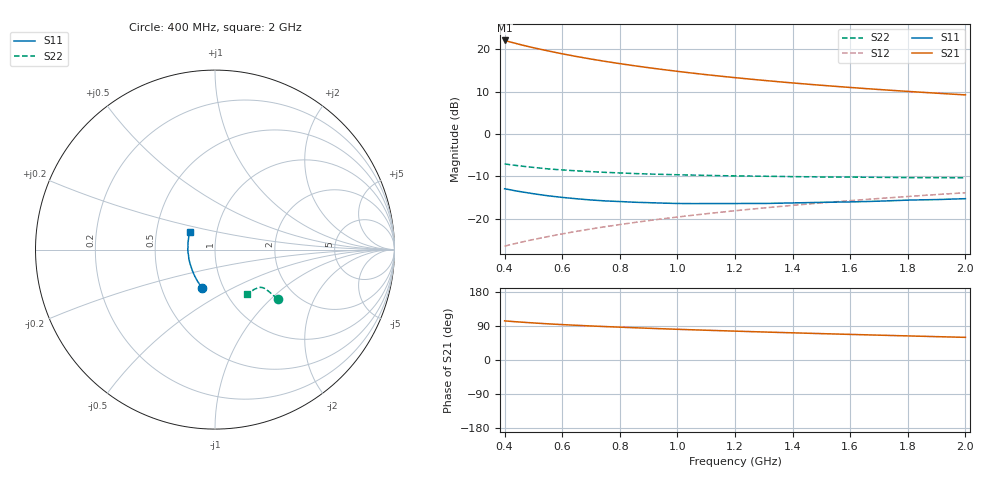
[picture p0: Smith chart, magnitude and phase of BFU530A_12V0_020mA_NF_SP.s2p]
! Filename:  P:\Prog\Test\Noise\ATS_data\Testdata_Net\06 Compressed Noise after Statistics\BFU530A_APG2013_33_A05_12p0V_020mA_NF_CM01_D.sf
! Date/Time: Tue 16/Apr/2013 15:11:00
! BFU530A_APG2013_33_A05_12p0V_1to25mA_NF_CM01_Bias7_R.sf
! Noise Parameter Data File
! BFU530A_APG2013_33_A05_12p0V_1to25mA_NF_CM01
! Date/time: Fri Apr 12 17:55:00 2013
! VAR V_out= 12.001000
! VAR I_out= 19.995000
! VAR V_in= 0.787500
! VAR I_in= 0.189800
! Device data file deembeded for feedlines and parallel
! Original file: \06 Compressed Noise after Statistics\BFU530A_APG2013_33_A05_12p0V_020mA_NF_CM01_R.sf
! Feed-files: PR017V01_150413_Feed1.s2p, PR017V01_150413_Feed2.s2p
! Parallel-file: PR017V01_150413_Par.s2p
# MHz S MA R 50
!  Freq-MHz  S11-mag  S11-arg  S21-mag  S21-arg  S12-mag  S12-arg  S22-mag  S22-arg
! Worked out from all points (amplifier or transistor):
!   37 points, 400 MHz to 2 GHz, reference 50 ohm
!   highest |S21| = 22.1 dB at 400 MHz (marker M1)
!   |S21| within 3 dB of that: start of sweep to 589.4 MHz
!   unconditionally stable (mu >= 1): 1.09 GHz to end of sweep
!   at 500 MHz: K = 0.91, MSG = 22.6 dB, |S12| = -24.9 dB
!   at 1.1 GHz: K = 1.00, MAG = 16.3 dB, |S12| = -18.8 dB
!   at 2 GHz: K = 1.00, MAG = 11.2 dB, |S12| = -13.9 dB
!   lowest NFmin = 1.08 dB at 420 MHz
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400  0.2256 -108.2  12.67 103.3  0.04747 70.6  0.4432 -38.2
420  0.2194 -110.9  12.14 102.0  0.0494 70.7  0.4334 -38.2
440  0.2127 -113.7  11.65 100.9  0.05122 70.9  0.4249 -38.2
460  0.2072 -116.0  11.2 99.8  0.05313 71.1  0.4174 -38.2
500  0.1972 -120.9  10.39 97.8  0.05685 71.4  0.4032 -38.1
550  0.1866 -127.0  9.552 95.4  0.06149 71.7  0.3873 -37.9
600  0.1785 -132.1  8.816 93.4  0.06627 71.9  0.3764 -37.9
650  0.1719 -137.3  8.19 91.6  0.07103 72.1  0.3672 -38.0
700  0.1664 -142.0  7.646 89.8  0.07579 72.2  0.3594 -38.0
750  0.1622 -146.6  7.169 88.2  0.0806 72.3  0.3523 -38.1
800  0.1595 -150.8  6.752 86.6  0.08539 72.3  0.3469 -38.3
850  0.1566 -155.3  6.379 85.1  0.09021 72.3  0.3412 -38.6
900  0.1547 -159.5  6.045 83.7  0.09505 72.2  0.3368 -38.9
950  0.1528 -163.2  5.746 82.4  0.09988 72.2  0.3335 -39.3
1050  0.1509 -170.1  5.229 79.8  0.1096 71.9  0.3272 -40.0
1100  0.1509 -173.5  5.005 78.6  0.1145 71.7  0.3249 -40.5
1200  0.1511 -179.7  4.614 76.2  0.1242 71.3  0.3203 -41.6
1350  0.1525 171.8  4.133 72.8  0.1389 70.5  0.3157 -43.5
1500  0.1561 164.1  3.749 69.6  0.1536 69.7  0.311 -45.6
1650  0.1594 157.5  3.436 66.5  0.1683 68.7  0.3086 -48.0
1750  0.1633 153.4  3.256 64.6  0.1781 68.0  0.3067 -49.6
2000  0.1724 144.6  2.888 59.8  0.2025 66.1  0.304 -54.2
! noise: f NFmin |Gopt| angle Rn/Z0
400  1.109  0.1852  -167.5  0.1002
460  1.084  0.1966  -166.5  0.0942
600  1.185  0.1737  -152.8  0.1134
800  1.171  0.2053  -157.1  0.0957
1000  1.179  0.2266  -152.7  0.0937
1200  1.221  0.2309  -148.7  0.1007
1400  1.223  0.2396  -142.2  0.1184
1600  1.245  0.2675  -135.4  0.1117
1800  1.25  0.288  -137.2  0.1045
2000  1.275  0.2852  -130.4  0.1191
